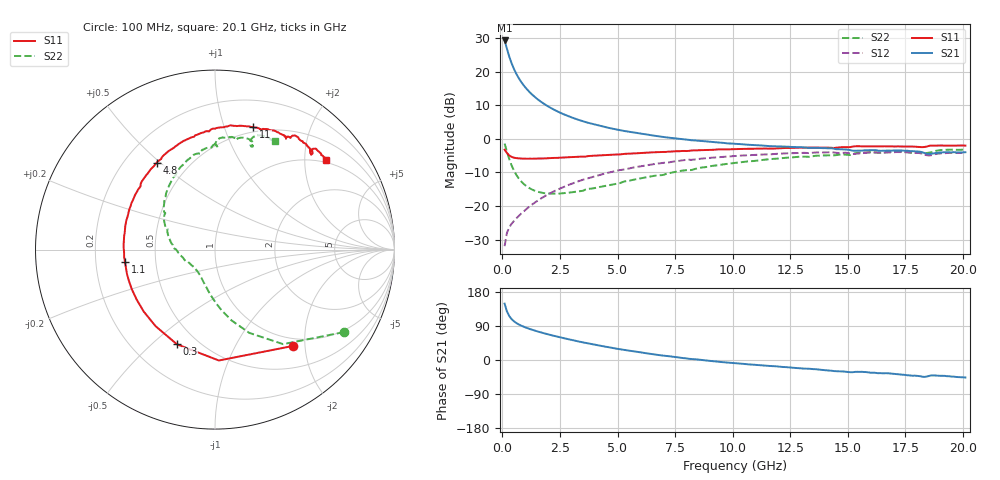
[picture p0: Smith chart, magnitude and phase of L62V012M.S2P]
!  Infineon Technologies AG
! BFR380L3 , PF131585-7, No.6, Th 09.10.01, soldered on pcb-board, measured with PP GSG850
!  Vce=2.0 V,  Ic=12.5 mA
! Common Emitter S-Parameters:  15. November 2001
#  GHz  S  MA  R  50
! f  S11  S21  S12  S22
! GHz  Mag  Ang  Mag  Ang  Mag  Ang  Mag  Ang
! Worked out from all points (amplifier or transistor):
!   201 points, 100 MHz to 20.1 GHz, reference 50 ohm
!   highest |S21| = 29.3 dB at 100 MHz (marker M1)
!   |S21| within 3 dB of that: start of sweep to 224.2 MHz
!   unconditionally stable (mu >= 1): 1.659 GHz to 4.652 GHz
!   at 3.4 GHz: K = 1.03, MAG = 7.9 dB, |S12| = -12.4 dB
!   at 10.1 GHz: K = 0.96, MSG = 1.8 dB, |S12| = -5.1 dB
!   at 20.1 GHz: K = 0.99, MSG = 0.1 dB, |S12| = -4.1 dB
!   S11 on the Smith chart (normalised r, x): 100 MHz: 0.86, -1.76; 300 MHz: 0.39, -0.60; 1.1 GHz: 0.33, -0.06; 4.8 GHz: 0.33, +0.49; 11 GHz: 0.45, +1.26; 20.1 GHz: 0.94, +2.54
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0.1  0.6896 -51.2  29.12 148.7  0.02536 67.2  0.8527 -32.6
0.2  0.6182 -88.0  21.99 128.3  0.03987 55.3  0.6492 -54.2
0.3  0.5686 -111.9  16.85 116.1  0.04822 51.1  0.5019 -67.6
0.4  0.5401 -127.8  13.42 108.1  0.05438 49.8  0.4055 -76.8
0.5  0.5261 -139.0  11.08 102.4  0.05975 50.5  0.3407 -83.8
0.6  0.5176 -147.7  9.391 98.0  0.06518 51.6  0.2952 -89.4
0.7  0.5133 -154.5  8.159 94.3  0.07065 52.9  0.2619 -94.2
0.8  0.5103 -160.0  7.195 91.2  0.07623 54.0  0.2372 -98.5
0.9  0.5089 -164.5  6.437 88.5  0.08177 55.1  0.2182 -102.2
1.1  0.5064 -172.3  5.326 83.8  0.09379 56.7  0.1927 -109.2
1.3  0.5068 -178.4  4.54 79.6  0.106 57.9  0.1757 -115.2
1.5  0.5098 176.2  3.964 75.9  0.1184 58.6  0.1652 -120.5
2  0.5169 165.2  3.023 67.5  0.1505 58.8  0.154 -132.2
2.7  0.5289 152.9  2.298 57.1  0.1953 56.9  0.1564 -146.1
3.5  0.5441 140.5  1.823 46.5  0.2467 53.3  0.169 -157.9
4.8  0.5818 124.0  1.417 31.6  0.3253 45.8  0.2104 -177.6
6.8  0.6359 103.1  1.09 12.9  0.4328 32.6  0.2878 157.4
10.1  0.7049 78.1  0.8441 -8.4  0.5561 11.2  0.4391 125.6
11  0.7146 72.6  0.8097 -12.9  0.5806 5.6  0.4721 117.6
13.5  0.7405 60.5  0.7394 -24.1  0.6228 -9.5  0.5532 98.1
16.8  0.7732 48.1  0.6688 -35.5  0.6281 -25.4  0.6395 77.1
20.1  0.7945 38.7  0.6334 -46.2  0.6211 -39.0  0.6931 61.0
